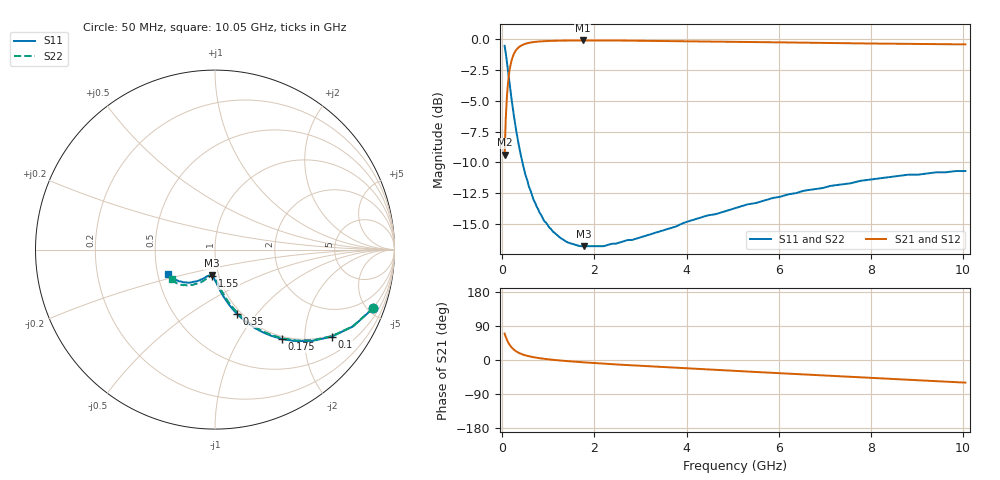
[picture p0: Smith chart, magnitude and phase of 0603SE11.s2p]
! AVX Thin Film Operation		Date: August 2001
! Description: Accu-P® Series, Thin Film, SMD, RF Capacitor
! Part Number: 06035J110FBT
! 50 MHz  -  10.05 GHz
! Serial Measurements
# mhz S db R 50
!	S11		S21		S12		S22
!	dB	Phase	dB	Phase	dB	Phase	dB	Phase
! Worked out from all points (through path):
!   401 points, 50 MHz to 10.05 GHz, reference 50 ohm
!   highest |S21| = -0.10 dB at 1.75 GHz (marker M1); lowest = -9.4 dB at 50 MHz (marker M2)
!   group delay of S21, straight-line fit = 20.6 ps
!   lowest |S11| = -16.8 dB at 1.775 GHz (marker M3), VSWR 1.34, Z = 46.2 - j13.5 ohm
!   |S11| at or under -10 dB: 437.1 MHz to end of sweep
!   |S22| runs from -16.8 to -0.5 dB; largest |S21 - S12| = 0
!   S11 on the Smith chart (normalised r, x): 50 MHz: 0.96, -5.42; 100 MHz: 0.96, -2.71; 175 MHz: 0.96, -1.56; 350 MHz: 0.95, -0.80; 1.55 GHz: 0.93, -0.28; 10.05 GHz: 0.57, -0.17
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50  -0.53 -20.3  -9.38 69.7  -9.38 69.7  -0.53 -20.2
100  -1.82 -36.7  -4.67 53.4  -4.67 53.4  -1.82 -36.4
125  -2.58 -43.2  -3.49 47.0  -3.49 47.0  -2.58 -42.8
175  -4.10 -53.1  -2.15 37.2  -2.15 37.2  -4.10 -52.5
200  -4.83 -56.9  -1.74 33.4  -1.74 33.4  -4.83 -56.3
250  -6.18 -63.0  -1.20 27.4  -1.20 27.4  -6.18 -62.2
350  -8.44 -71.1  -0.68 19.4  -0.68 19.4  -8.44 -70.1
450  -10.21 -76.2  -0.44 14.3  -0.44 14.3  -10.21 -75.0
550  -11.56 -79.9  -0.32 10.7  -0.32 10.7  -11.56 -78.4
700  -13.19 -83.9  -0.22 6.9  -0.22 6.9  -13.19 -82.0
850  -14.31 -86.8  -0.17 4.1  -0.17 4.1  -14.31 -84.7
1150  -15.77 -91.3  -0.12 -0.1  -0.12 -0.1  -15.77 -88.6
1550  -16.64 -95.6  -0.10 -4.2  -0.10 -4.2  -16.64 -92.4
1725  -16.80 -97.2  -0.10 -5.8  -0.10 -5.8  -16.80 -94.0
1750  -16.80 -97.4  -0.10 -6.1  -0.10 -6.1  -16.80 -94.1
1775  -16.80 -97.6  -0.10 -6.3  -0.10 -6.3  -16.80 -94.3
2475  -16.58 -103.2  -0.10 -11.8  -0.10 -11.8  -16.58 -99.5
3400  -15.62 -109.9  -0.13 -18.2  -0.13 -18.2  -15.53 -105.9
5050  -13.72 -120.8  -0.20 -28.9  -0.20 -28.9  -13.66 -116.4
6725  -12.20 -132.0  -0.29 -39.2  -0.29 -39.2  -12.20 -126.0
8400  -11.19 -142.2  -0.36 -49.6  -0.36 -49.6  -11.19 -136.1
10050  -10.70 -152.8  -0.41 -59.5  -0.41 -59.5  -10.70 -145.6
